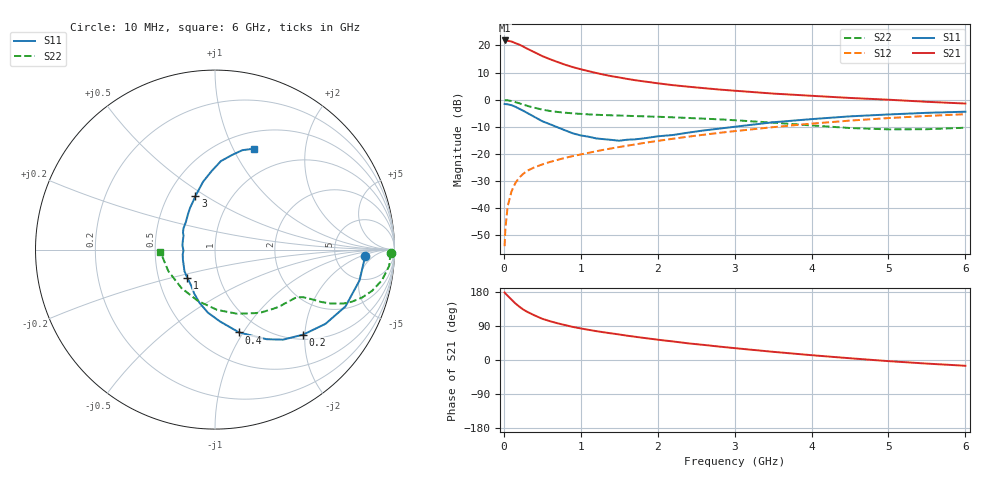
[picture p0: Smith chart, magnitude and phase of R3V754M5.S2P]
! SIEMENS Small Signal Semiconductors
! BFR181
! Si NPN RF Bipolar Junction Transistor in SOT23
! VCE = 0.75 V  IC = 4.5 mA
! Common Emitter S-Parameters:  May  1996
# GHz  S  MA  R  50
!  f  S11  S21  S12  S22
! GHz  MAG  ANG  MAG  ANG  MAG  ANG  MAG  ANG
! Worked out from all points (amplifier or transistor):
!   36 points, 10 MHz to 6 GHz, reference 50 ohm
!   highest |S21| = 21.9 dB at 10 MHz (marker M1)
!   |S21| within 3 dB of that: start of sweep to 300.9 MHz
!   unconditionally stable (mu >= 1): 893.2 MHz to 3.431 GHz
!   at 250 MHz: K = 0.43, MSG = 23.5 dB, |S12| = -27.4 dB
!   at 1.4 GHz: K = 1.12, MAG = 11.2 dB, |S12| = -17.9 dB
!   at 6 GHz: K = 0.92, MSG = 2.0 dB, |S12| = -5.3 dB
!   S11 on the Smith chart (normalised r, x): 10 MHz: 11, -3; 200 MHz: 1.11, -1.96; 400 MHz: 0.80, -0.96; 1 GHz: 0.70, -0.23; 3 GHz: 0.68, +0.45; 6 GHz: 0.68, +1.21
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0.01  0.8371 -2.6  12.38 178.0  0.002 88.5  0.9828 -1.1
0.02  0.8317 -4.9  12.16 175.7  0.0042 88.8  0.9766 -2.2
0.05  0.8236 -12.0  12.21 169.4  0.0109 83.2  0.9746 -5.4
0.1  0.793 -23.5  11.84 159.3  0.0205 76.9  0.9457 -10.4
0.15  0.7417 -33.9  11.06 149.3  0.0292 71.7  0.9049 -14.7
0.2  0.6826 -43.9  10.4 141.0  0.0368 68.5  0.8612 -18.1
0.25  0.6292 -52.9  9.588 133.5  0.0428 64.8  0.8149 -20.9
0.3  0.5758 -60.1  8.775 127.5  0.0487 63.0  0.7756 -22.8
0.4  0.4805 -73.8  7.486 117.6  0.057 59.9  0.7109 -25.0
0.5  0.4015 -86.0  6.374 108.7  0.0642 58.6  0.6574 -26.3
0.6  0.3535 -96.4  5.585 102.4  0.0713 58.2  0.6204 -26.9
0.8  0.2717 -115.1  4.406 91.9  0.0851 58.1  0.576 -27.9
1  0.2198 -134.7  3.646 83.3  0.0982 59.4  0.5482 -28.9
1.1  0.2084 -144.7  3.364 79.7  0.105 59.7  0.5371 -29.6
1.3  0.1875 -162.3  2.898 73.1  0.1197 60.2  0.5216 -31.1
1.6  0.1831 172.7  2.426 64.2  0.1419 60.2  0.5057 -34.3
2.2  0.224 136.3  1.855 48.9  0.1912 58.6  0.4741 -42.6
3  0.3176 110.1  1.467 31.3  0.2637 53.6  0.4191 -57.6
3.5  0.3844 99.9  1.299 21.6  0.3124 49.3  0.3783 -70.9
4.5  0.4941 86.2  1.079 4.6  0.4125 38.0  0.3011 -108.6
5.5  0.574 74.7  0.916 -9.5  0.5027 24.9  0.2863 -155.2
6  0.6018 69.1  0.851 -15.2  0.5417 17.7  0.305 -177.8
